| IBIS file stm32u535_545_wlcsp72.ibs
[IBIS ver] 4.2
[File name] stm32u535_545_wlcsp72.ibs
[File Rev] rev1.0
[Date]  11-09-2023
[Source] Data Created at STMicroelectronics
[Notes]  File originated from ELDO simulations.
[Disclaimer]  This information is for modeling purpose only and is
   not guaranteed. The information is subject to change without
   notice.
[Copyright] Copyright 2023 STMicroelectronics Inc.
|   Component stm32u535_545_wlcsp72
[Component] stm32u535_545_wlcsp72
[Manufacturer] STMicroelectronics
[Package]
| variable   typ   min   max
R_pkg  0  NA  NA
L_pkg  0  NA  NA
C_pkg  0  NA  NA
[Pin]   signal_name   model_name
A2  VDD  power
A4  PG10  io8_100m_hslv_ft
A6  PG14  io8_100m_hslv_i2c_ft
A8  VDDIO2  power
A10  PB4  io8_100m_i2c_ft
A12  PH3-BOOT0  io8_100m_ft
A14  VDD11  nc
A16  VDD  power
B1  VDDUSB  power
B3  VSS  gnd
B5  PG9  io8_100m_hslv_ft
B7  VSS  gnd
B9  PG15  io8_100m_hslv_ft
B11  PB6  io8_100m_i2c_ft
B13  VSS  gnd
B15  VBAT  power
C2  PA11  io8_usb_ft
C4  PA12  io8_usb_ft
C6  PG11  io8_100m_hslv_ft
C8  PG13  io8_100m_hslv_i2c_ft
C10  PB3  io8_100m_i2c_ft
C12  PB8  io8_100m_hslv_i2c_ft
C14  PC13  io8_100m_ft_v33
C16  PC14-OSC32_IN   io8_100m_tamp_ft
D1  VDDIO2  power
D3  VSS  gnd
D5  PA13  io8_100m_ft
D7  PA15  io8_100m_ft
D9  PG12  io8_100m_hslv_ft
D11  PB5  io8_166m_hslv_ft
D13  PB7  io8_166m_hslv_i2c_ft
D15  PC15-OSC32_OUT  io8_100m_tamp_ft
E2  PG8  io8_100m_i2c_ft
E4  PA8  io8_166m_hslv_ft
E6  PA10  io8_100m_ft
E8  PA14  io8_100m_ft
E10  PA5  io8_100m_ft
E12  PA1  io8_100m_hslv_tamp_ft
E14  NRST  nc
E16  PH0-OSC_IN  io8_100m_ft
F1  PG4  io8_100m_hslv_ft
F3  PG5  io8_100m_hslv_ft
F5  PG6  io8_100m_hslv_ft
F7  PG7  io8_100m_hslv_i2c_ft
F9  PA9  io8_100m_ft
F11  PA2  io8_100m_hslv_ft
F13  PC1  io8_166m_hslv_i2c_ft
F15  PH1-OSC_OUT  io8_100m_ft
G2  PB14  io8_100m_i2c_ft
G4  PB13  io8_100m_i2c_ft
G6  PG2  io8_100m_hslv_ft
G8  PB1  io8_100m_hslv_ft
G10  PB0  io8_100m_hslv_ft
G12  PA3  io8_166m_hslv_ft
G14  VDDA  power
G16  VSSA  nc
H1  PB15  io8_100m_ft
H3  VSS  gnd
H5  VSSSMPS  nc
H7  PG3  io8_100m_hslv_ft
H9  PB10  io8_166m_hslv_i2c_ft
H11  PA6  io8_100m_hslv_ft
H13  PA4  io8_100m_hslv_ft
H15  PA0  io8_100m_hslv_tamp_ft
J2  VDD  power
J4  VDD11  nc
J6  VDDSMPS  nc
J8  VLXSMPS  nc
J10  PB2  io8_100m_hslv_tamp_ft
J12  PA7  io8_100m_hslv_i2c_ft
J14  VDD  power
J16  VSS  gnd
[Package Model]   455-wlcsp-72-100mhz-230421
[Pin Mapping]   pulldown_ref   pullup_ref   | Comment
A2  nc  vddiom
A4  gndio  vddiom
A6  gndio  vddiom  | Depending on IO usage
| A6  gndio  vddios  | Depending on IO usage
A8  nc  vddios
A10  gndio  vddiom
A12  gndio  vddiom
A14  nc  nc
A16  nc  vddiom
B1  nc  vddusb
B3  gndio  nc
B5  gndio  vddiom  | Depending on IO usage
| B5  gndio  vddios  | Depending on IO usage
B7  gndio  nc
B9  gndio  vddiom  | Depending on IO usage
| B9  gndio  vddios  | Depending on IO usage
B11  gndio  vddiom
B13  gndio  nc
B15  nc  vsw
C2  gndio  vddiom  | Depending on IO usage
| C2  gndio  vddusb  | Depending on IO usage
C4  gndio  vddiom  | Depending on IO usage
| C4  gndio  vddusb  | Depending on IO usage
C6  gndio  vddiom  | Depending on IO usage
| C6  gndio  vddios  | Depending on IO usage
C8  gndio  vddiom  | Depending on IO usage
| C8  gndio  vddios  | Depending on IO usage
C10  gndio  vddiom
C12  gndio  vddiom
C14  gndio  vddiom  | Depending on IO usage
| C14  gndio  vsw  | Depending on IO usage
C16  gndio  vddiom  | Depending on IO usage
| C16  gndio  vsw  | Depending on IO usage
D1  nc  vddios
D3  gndio  nc
D5  gndio  vddiom  | Depending on IO usage
| D5  gndio  vddusb  | Depending on IO usage
D7  gndio  vddiom
D9  gndio  vddiom  | Depending on IO usage
| D9  gndio  vddios  | Depending on IO usage
D11  gndio  vddiom
D13  gndio  vddiom
D15  gndio  vddiom  | Depending on IO usage
| D15  gndio  vsw  | Depending on IO usage
E2  gndio  vddiom  | Depending on IO usage
| E2  gndio  vddios  | Depending on IO usage
E4  gndio  vddiom
E6  gndio  vddiom  | Depending on IO usage
| E6  gndio  vddusb  | Depending on IO usage
E8  gndio  vddiom
E10  gndio  vddiom
E12  gndio  vddiom
E14  nc   nc
E16  gndio  vddiom
F1  gndio  vddiom  | Depending on IO usage
| F1  gndio  vddios  | Depending on IO usage
F3  gndio  vddiom  | Depending on IO usage
| F3  gndio  vddios  | Depending on IO usage
F5  gndio  vddiom  | Depending on IO usage
| F5  gndio  vddios  | Depending on IO usage
F7  gndio  vddiom  | Depending on IO usage
| F7  gndio  vddios  | Depending on IO usage
F9  gndio  vddiom  | Depending on IO usage
| F9  gndio  vddusb  | Depending on IO usage
F11  gndio  vddiom
F13  gndio  vddiom
F15  gndio  vddiom
G2  gndio  vddiom
G4  gndio  vddiom
G6  gndio  vddiom  | Depending on IO usage
| G6  gndio  vddios  | Depending on IO usage
G8  gndio  vddiom
G10  gndio  vddiom
G12  gndio  vddiom
G14  nc  vddiom
G16  nc  nc
H1  gndio  vddiom
H3  gndio  nc
H5  nc  nc
H7  gndio  vddiom  | Depending on IO usage
| H7  gndio  vddios  | Depending on IO usage
H9  gndio  vddiom
H11  gndio  vddiom
H13  gndio  vddiom
H15  gndio  vddiom
J2  nc  vddiom
J4  nc  nc
J6  nc  nc
J8  nc  nc
J10  gndio  vddiom
J12  gndio  vddiom
J14  nc  vddiom
J16  gndio  nc
[Model Selector] io8_100m_ft
io8_100m_ft_hs_1v2  "IO8_FT 100MHz high speed @ 1.2V"
io8_100m_ft_fs_1v2  "IO8_FT 100MHz fast speed @ 1.2V"
io8_100m_ft_fs_pd_1v2  "IO8_FT 100MHz fast speed @ 1.2V pulldown"
io8_100m_ft_ms_1v2  "IO8_FT 100MHz med speed @ 1.2V"
io8_100m_ft_ms_pd_1v2  "IO8_FT 100MHz med speed @ 1.2V pulldown"
io8_100m_ft_ls_1v2  "IO8_FT 100MHz low speed @ 1.2V"
io8_100m_ft_ls_pd_1v2  "IO8_FT 100MHz low speed @ 1.2V pulldown"
io8_100m_ft_hs_1v8  "IO8_FT 100MHz high speed @ 1.8V"
io8_100m_ft_hs_pd_1v8  "IO8_FT 100MHz high speed @ 1.8V pulldown"
io8_100m_ft_fs_1v8  "IO8_FT 100MHz fast speed @ 1.8V"
io8_100m_ft_fs_pd_1v8  "IO8_FT 100MHz fast speed @ 1.8V pulldown"
io8_100m_ft_ms_1v8  "IO8_FT 100MHz med speed @ 1.8V"
io8_100m_ft_ms_pd_1v8  "IO8_FT 100MHz med speed @ 1.8V pulldown"
io8_100m_ft_ls_1v8  "IO8_FT 100MHz low speed @ 1.8V"
io8_100m_ft_ls_pd_1v8  "IO8_FT 100MHz low speed @ 1.8V pulldown"
io8_100m_ft_hs_3v3  "IO8_FT 100MHz high speed @ 3.3V"
io8_100m_ft_hs_pd_3v3  "IO8_FT 100MHz high speed @ 3.3V pulldown"
io8_100m_ft_fs_3v3  "IO8_FT 100MHz fast speed @ 3.3V"
io8_100m_ft_fs_pd_3v3  "IO8_FT 100MHz fast speed @ 3.3V pulldown"
io8_100m_ft_ms_3v3  "IO8_FT 100MHz med speed @ 3.3V"
io8_100m_ft_ms_pd_3v3  "IO8_FT 100MHz med speed @ 3.3V pulldown"
io8_100m_ft_ls_3v3  "IO8_FT 100MHz low speed @ 3.3V"
io8_100m_ft_ls_pd_3v3  "IO8_FT 100MHz low speed @ 3.3V pulldown"
[Model Selector] io8_100m_hslv_ft
io8_100m_ft_hs_1v2  "IO8_FT 100MHz high speed @ 1.2V"
io8_100m_ft_hs_pu_1v2  "IO8_FT 100MHz high speed @ 1.2V pullup"
io8_100m_ft_hs_pd_1v2  "IO8_FT 100MHz high speed @ 1.2V pulldown"
io8_100m_ft_fs_1v2  "IO8_FT 100MHz fast speed @ 1.2V"
io8_100m_ft_fs_pu_1v2  "IO8_FT 100MHz fast speed @ 1.2V pullup"
io8_100m_ft_fs_pd_1v2  "IO8_FT 100MHz fast speed @ 1.2V pulldown"
io8_100m_ft_ms_1v2  "IO8_FT 100MHz med speed @ 1.2V"
io8_100m_ft_ms_pu_1v2  "IO8_FT 100MHz med speed @ 1.2V pullup"
io8_100m_ft_ms_pd_1v2  "IO8_FT 100MHz med speed @ 1.2V pulldown"
io8_100m_ft_ls_1v2  "IO8_FT 100MHz low speed @ 1.2V"
io8_100m_ft_ls_pu_1v2  "IO8_FT 100MHz low speed @ 1.2V pullup"
io8_100m_ft_ls_pd_1v2  "IO8_FT 100MHz low speed @ 1.2V pulldown"
io8_100m_ft_hs_1v8  "IO8_FT 100MHz high speed @ 1.8V"
io8_100m_ft_hs_pu_1v8  "IO8_FT 100MHz high speed @ 1.8V pullup"
io8_100m_ft_hs_pd_1v8  "IO8_FT 100MHz high speed @ 1.8V pulldown"
io8_100m_ft_fs_1v8  "IO8_FT 100MHz fast speed @ 1.8V"
io8_100m_ft_fs_pu_1v8  "IO8_FT 100MHz fast speed @ 1.8V pullup"
io8_100m_ft_fs_pd_1v8  "IO8_FT 100MHz fast speed @ 1.8V pulldown"
io8_100m_ft_ms_1v8  "IO8_FT 100MHz med speed @ 1.8V"
io8_100m_ft_ms_pu_1v8  "IO8_FT 100MHz med speed @ 1.8V pullup"
io8_100m_ft_ms_pd_1v8  "IO8_FT 100MHz med speed @ 1.8V pulldown"
io8_100m_ft_ls_1v8  "IO8_FT 100MHz low speed @ 1.8V"
io8_100m_ft_ls_pu_1v8  "IO8_FT 100MHz low speed @ 1.8V pullup"
io8_100m_ft_ls_pd_1v8  "IO8_FT 100MHz low speed @ 1.8V pulldown"
io8_100m_ft_hs_3v3  "IO8_FT 100MHz high speed @ 3.3V"
io8_100m_ft_hs_pu_3v3  "IO8_FT 100MHz high speed @ 3.3V pullup"
io8_100m_ft_hs_pd_3v3  "IO8_FT 100MHz high speed @ 3.3V pulldown"
io8_100m_ft_fs_3v3  "IO8_FT 100MHz fast speed @ 3.3V"
io8_100m_ft_fs_pu_3v3  "IO8_FT 100MHz fast speed @ 3.3V pullup"
io8_100m_ft_fs_pd_3v3  "IO8_FT 100MHz fast speed @ 3.3V pulldown"
io8_100m_ft_ms_3v3  "IO8_FT 100MHz med speed @ 3.3V"
io8_100m_ft_ms_pu_3v3  "IO8_FT 100MHz med speed @ 3.3V pullup"
io8_100m_ft_ms_pd_3v3  "IO8_FT 100MHz med speed @ 3.3V pulldown"
io8_100m_ft_ls_3v3  "IO8_FT 100MHz low speed @ 3.3V"
io8_100m_ft_ls_pu_3v3  "IO8_FT 100MHz low speed @ 3.3V pullup"
io8_100m_ft_ls_pd_3v3  "IO8_FT 100MHz low speed @ 3.3V pulldown"
io8_100m_hslv_ft_hs_1v2  "IO8_FT 100MHz HSLV high speed @ 1.2V"
io8_100m_hslv_ft_hs_pu_1v2  "IO8_FT 100MHz HSLV high speed @ 1.2V pullup"
io8_100m_hslv_ft_hs_pd_1v2  "IO8_FT 100MHz HSLV high speed @ 1.2V pulldown"
io8_100m_hslv_ft_fs_1v2  "IO8_FT 100MHz HSLV fast speed @ 1.2V"
io8_100m_hslv_ft_fs_pu_1v2  "IO8_FT 100MHz HSLV fast speed @ 1.2V pullup"
io8_100m_hslv_ft_fs_pd_1v2  "IO8_FT 100MHz HSLV fast speed @ 1.2V pulldown"
io8_100m_hslv_ft_ms_1v2  "IO8_FT 100MHz HSLV med speed @ 1.2V"
io8_100m_hslv_ft_ms_pu_1v2  "IO8_FT 100MHz HSLV med speed @ 1.2V pullup"
io8_100m_hslv_ft_ms_pd_1v2  "IO8_FT 100MHz HSLV med speed @ 1.2V pulldown"
io8_100m_hslv_ft_ls_1v2  "IO8_FT 100MHz HSLV low speed @ 1.2V"
io8_100m_hslv_ft_ls_pu_1v2  "IO8_FT 100MHz HSLV low speed @ 1.2V pullup"
io8_100m_hslv_ft_ls_pd_1v2  "IO8_FT 100MHz HSLV low speed @ 1.2V pulldown"
io8_100m_hslv_ft_hs_1v8  "IO8_FT 100MHz HSLV high speed @ 1.8V"
io8_100m_hslv_ft_hs_pu_1v8  "IO8_FT 100MHz HSLV high speed @ 1.8V pullup"
io8_100m_hslv_ft_hs_pd_1v8  "IO8_FT 100MHz HSLV high speed @ 1.8V pulldown"
io8_100m_hslv_ft_fs_1v8  "IO8_FT 100MHz HSLV fast speed @ 1.8V"
io8_100m_hslv_ft_fs_pu_1v8  "IO8_FT 100MHz HSLV fast speed @ 1.8V pullup"
io8_100m_hslv_ft_fs_pd_1v8  "IO8_FT 100MHz HSLV fast speed @ 1.8V pulldown"
io8_100m_hslv_ft_ms_1v8  "IO8_FT 100MHz HSLV med speed @ 1.8V"
io8_100m_hslv_ft_ms_pu_1v8  "IO8_FT 100MHz HSLV med speed @ 1.8V pullup"
io8_100m_hslv_ft_ms_pd_1v8  "IO8_FT 100MHz HSLV med speed @ 1.8V pulldown"
io8_100m_hslv_ft_ls_1v8  "IO8_FT 100MHz HSLV low speed @ 1.8V"
io8_100m_hslv_ft_ls_pu_1v8  "IO8_FT 100MHz HSLV low speed @ 1.8V pullup"
io8_100m_hslv_ft_ls_pd_1v8  "IO8_FT 100MHz HSLV low speed @ 1.8V pulldown"
io8_100m_hslv_ft_hs_2v5  "IO8_FT 100MHz HSLV high speed @ 2.5V"
io8_100m_hslv_ft_hs_pu_2v5  "IO8_FT 100MHz HSLV high speed @ 2.5V pullup"
io8_100m_hslv_ft_hs_pd_2v5  "IO8_FT 100MHz HSLV high speed @ 2.5V pulldown"
io8_100m_hslv_ft_fs_2v5  "IO8_FT 100MHz HSLV fast speed @ 2.5V"
io8_100m_hslv_ft_fs_pu_2v5  "IO8_FT 100MHz HSLV fast speed @ 2.5V pullup"
io8_100m_hslv_ft_fs_pd_2v5  "IO8_FT 100MHz HSLV fast speed @ 2.5V pulldown"
io8_100m_hslv_ft_ms_2v5  "IO8_FT 100MHz HSLV med speed @ 2.5V"
io8_100m_hslv_ft_ms_pu_2v5  "IO8_FT 100MHz HSLV med speed @ 2.5V pullup"
io8_100m_hslv_ft_ms_pd_2v5  "IO8_FT 100MHz HSLV med speed @ 2.5V pulldown"
io8_100m_hslv_ft_ls_2v5  "IO8_FT 100MHz HSLV low speed @ 2.5V"
io8_100m_hslv_ft_ls_pu_2v5  "IO8_FT 100MHz HSLV low speed @ 2.5V pullup"
io8_100m_hslv_ft_ls_pd_2v5  "IO8_FT 100MHz HSLV low speed @ 2.5V pulldown"
[Model Selector] io8_100m_hslv_i2c_ft
io8_100m_ft_hs_1v2  "IO8_FT 100MHz high speed @ 1.2V"
io8_100m_ft_hs_pu_1v2  "IO8_FT 100MHz high speed @ 1.2V pullup"
io8_100m_ft_hs_pd_1v2  "IO8_FT 100MHz high speed @ 1.2V pulldown"
io8_100m_ft_fs_1v2  "IO8_FT 100MHz fast speed @ 1.2V"
io8_100m_ft_fs_pu_1v2  "IO8_FT 100MHz fast speed @ 1.2V pullup"
io8_100m_ft_fs_pd_1v2  "IO8_FT 100MHz fast speed @ 1.2V pulldown"
io8_100m_ft_ms_1v2  "IO8_FT 100MHz med speed @ 1.2V"
io8_100m_ft_ms_pu_1v2  "IO8_FT 100MHz med speed @ 1.2V pullup"
io8_100m_ft_ms_pd_1v2  "IO8_FT 100MHz med speed @ 1.2V pulldown"
io8_100m_ft_ls_1v2  "IO8_FT 100MHz low speed @ 1.2V"
io8_100m_ft_ls_pu_1v2  "IO8_FT 100MHz low speed @ 1.2V pullup"
io8_100m_ft_ls_pd_1v2  "IO8_FT 100MHz low speed @ 1.2V pulldown"
io8_100m_ft_hs_1v8  "IO8_FT 100MHz high speed @ 1.8V"
io8_100m_ft_hs_pu_1v8  "IO8_FT 100MHz high speed @ 1.8V pullup"
io8_100m_ft_hs_pd_1v8  "IO8_FT 100MHz high speed @ 1.8V pulldown"
io8_100m_ft_fs_1v8  "IO8_FT 100MHz fast speed @ 1.8V"
io8_100m_ft_fs_pu_1v8  "IO8_FT 100MHz fast speed @ 1.8V pullup"
io8_100m_ft_fs_pd_1v8  "IO8_FT 100MHz fast speed @ 1.8V pulldown"
io8_100m_ft_ms_1v8  "IO8_FT 100MHz med speed @ 1.8V"
io8_100m_ft_ms_pu_1v8  "IO8_FT 100MHz med speed @ 1.8V pullup"
io8_100m_ft_ms_pd_1v8  "IO8_FT 100MHz med speed @ 1.8V pulldown"
io8_100m_ft_ls_1v8  "IO8_FT 100MHz low speed @ 1.8V"
io8_100m_ft_ls_pu_1v8  "IO8_FT 100MHz low speed @ 1.8V pullup"
io8_100m_ft_ls_pd_1v8  "IO8_FT 100MHz low speed @ 1.8V pulldown"
io8_100m_ft_hs_3v3  "IO8_FT 100MHz high speed @ 3.3V"
io8_100m_ft_hs_pu_3v3  "IO8_FT 100MHz high speed @ 3.3V pullup"
io8_100m_ft_hs_pd_3v3  "IO8_FT 100MHz high speed @ 3.3V pulldown"
io8_100m_ft_fs_3v3  "IO8_FT 100MHz fast speed @ 3.3V"
io8_100m_ft_fs_pu_3v3  "IO8_FT 100MHz fast speed @ 3.3V pullup"
io8_100m_ft_fs_pd_3v3  "IO8_FT 100MHz fast speed @ 3.3V pulldown"
io8_100m_ft_ms_3v3  "IO8_FT 100MHz med speed @ 3.3V"
io8_100m_ft_ms_pu_3v3  "IO8_FT 100MHz med speed @ 3.3V pullup"
io8_100m_ft_ms_pd_3v3  "IO8_FT 100MHz med speed @ 3.3V pulldown"
io8_100m_ft_ls_3v3  "IO8_FT 100MHz low speed @ 3.3V"
io8_100m_ft_ls_pu_3v3  "IO8_FT 100MHz low speed @ 3.3V pullup"
io8_100m_ft_ls_pd_3v3  "IO8_FT 100MHz low speed @ 3.3V pulldown"
io8_100m_hslv_ft_hs_1v2  "IO8_FT 100MHz HSLV high speed @ 1.2V"
io8_100m_hslv_ft_hs_pu_1v2  "IO8_FT 100MHz HSLV high speed @ 1.2V pullup"
io8_100m_hslv_ft_hs_pd_1v2  "IO8_FT 100MHz HSLV high speed @ 1.2V pulldown"
io8_100m_hslv_ft_fs_1v2  "IO8_FT 100MHz HSLV fast speed @ 1.2V"
io8_100m_hslv_ft_fs_pu_1v2  "IO8_FT 100MHz HSLV fast speed @ 1.2V pullup"
io8_100m_hslv_ft_fs_pd_1v2  "IO8_FT 100MHz HSLV fast speed @ 1.2V pulldown"
io8_100m_hslv_ft_ms_1v2  "IO8_FT 100MHz HSLV med speed @ 1.2V"
io8_100m_hslv_ft_ms_pu_1v2  "IO8_FT 100MHz HSLV med speed @ 1.2V pullup"
io8_100m_hslv_ft_ms_pd_1v2  "IO8_FT 100MHz HSLV med speed @ 1.2V pulldown"
io8_100m_hslv_ft_ls_1v2  "IO8_FT 100MHz HSLV low speed @ 1.2V"
io8_100m_hslv_ft_ls_pu_1v2  "IO8_FT 100MHz HSLV low speed @ 1.2V pullup"
io8_100m_hslv_ft_ls_pd_1v2  "IO8_FT 100MHz HSLV low speed @ 1.2V pulldown"
io8_100m_hslv_ft_hs_1v8  "IO8_FT 100MHz HSLV high speed @ 1.8V"
io8_100m_hslv_ft_hs_pu_1v8  "IO8_FT 100MHz HSLV high speed @ 1.8V pullup"
io8_100m_hslv_ft_hs_pd_1v8  "IO8_FT 100MHz HSLV high speed @ 1.8V pulldown"
io8_100m_hslv_ft_fs_1v8  "IO8_FT 100MHz HSLV fast speed @ 1.8V"
io8_100m_hslv_ft_fs_pu_1v8  "IO8_FT 100MHz HSLV fast speed @ 1.8V pullup"
io8_100m_hslv_ft_fs_pd_1v8  "IO8_FT 100MHz HSLV fast speed @ 1.8V pulldown"
io8_100m_hslv_ft_ms_1v8  "IO8_FT 100MHz HSLV med speed @ 1.8V"
io8_100m_hslv_ft_ms_pu_1v8  "IO8_FT 100MHz HSLV med speed @ 1.8V pullup"
io8_100m_hslv_ft_ms_pd_1v8  "IO8_FT 100MHz HSLV med speed @ 1.8V pulldown"
io8_100m_hslv_ft_ls_1v8  "IO8_FT 100MHz HSLV low speed @ 1.8V"
io8_100m_hslv_ft_ls_pu_1v8  "IO8_FT 100MHz HSLV low speed @ 1.8V pullup"
io8_100m_hslv_ft_ls_pd_1v8  "IO8_FT 100MHz HSLV low speed @ 1.8V pulldown"
io8_100m_hslv_ft_hs_2v5  "IO8_FT 100MHz HSLV high speed @ 2.5V"
io8_100m_hslv_ft_hs_pu_2v5  "IO8_FT 100MHz HSLV high speed @ 2.5V pullup"
io8_100m_hslv_ft_hs_pd_2v5  "IO8_FT 100MHz HSLV high speed @ 2.5V pulldown"
io8_100m_hslv_ft_fs_2v5  "IO8_FT 100MHz HSLV fast speed @ 2.5V"
io8_100m_hslv_ft_fs_pu_2v5  "IO8_FT 100MHz HSLV fast speed @ 2.5V pullup"
io8_100m_hslv_ft_fs_pd_2v5  "IO8_FT 100MHz HSLV fast speed @ 2.5V pulldown"
io8_100m_hslv_ft_ms_2v5  "IO8_FT 100MHz HSLV med speed @ 2.5V"
io8_100m_hslv_ft_ms_pu_2v5  "IO8_FT 100MHz HSLV med speed @ 2.5V pullup"
io8_100m_hslv_ft_ms_pd_2v5  "IO8_FT 100MHz HSLV med speed @ 2.5V pulldown"
io8_100m_hslv_ft_ls_2v5  "IO8_FT 100MHz HSLV low speed @ 2.5V"
io8_100m_hslv_ft_ls_pu_2v5  "IO8_FT 100MHz HSLV low speed @ 2.5V pullup"
io8_100m_hslv_ft_ls_pd_2v5  "IO8_FT 100MHz HSLV low speed @ 2.5V pulldown"
[Model Selector] io8_100m_hslv_tamp_ft
io8_100m_ft_hs_1v2  "IO8_FT 100MHz high speed @ 1.2V"
io8_100m_ft_hs_pu_1v2  "IO8_FT 100MHz high speed @ 1.2V pullup"
io8_100m_ft_hs_pd_1v2  "IO8_FT 100MHz high speed @ 1.2V pulldown"
io8_100m_ft_fs_1v2  "IO8_FT 100MHz fast speed @ 1.2V"
io8_100m_ft_fs_pu_1v2  "IO8_FT 100MHz fast speed @ 1.2V pullup"
io8_100m_ft_fs_pd_1v2  "IO8_FT 100MHz fast speed @ 1.2V pulldown"
io8_100m_ft_ms_1v2  "IO8_FT 100MHz med speed @ 1.2V"
io8_100m_ft_ms_pu_1v2  "IO8_FT 100MHz med speed @ 1.2V pullup"
io8_100m_ft_ms_pd_1v2  "IO8_FT 100MHz med speed @ 1.2V pulldown"
io8_100m_ft_ls_1v2  "IO8_FT 100MHz low speed @ 1.2V"
io8_100m_ft_ls_pu_1v2  "IO8_FT 100MHz low speed @ 1.2V pullup"
io8_100m_ft_ls_pd_1v2  "IO8_FT 100MHz low speed @ 1.2V pulldown"
io8_100m_ft_hs_1v8  "IO8_FT 100MHz high speed @ 1.8V"
io8_100m_ft_hs_pu_1v8  "IO8_FT 100MHz high speed @ 1.8V pullup"
io8_100m_ft_hs_pd_1v8  "IO8_FT 100MHz high speed @ 1.8V pulldown"
io8_100m_ft_fs_1v8  "IO8_FT 100MHz fast speed @ 1.8V"
io8_100m_ft_fs_pu_1v8  "IO8_FT 100MHz fast speed @ 1.8V pullup"
io8_100m_ft_fs_pd_1v8  "IO8_FT 100MHz fast speed @ 1.8V pulldown"
io8_100m_ft_ms_1v8  "IO8_FT 100MHz med speed @ 1.8V"
io8_100m_ft_ms_pu_1v8  "IO8_FT 100MHz med speed @ 1.8V pullup"
io8_100m_ft_ms_pd_1v8  "IO8_FT 100MHz med speed @ 1.8V pulldown"
io8_100m_ft_ls_1v8  "IO8_FT 100MHz low speed @ 1.8V"
io8_100m_ft_ls_pu_1v8  "IO8_FT 100MHz low speed @ 1.8V pullup"
io8_100m_ft_ls_pd_1v8  "IO8_FT 100MHz low speed @ 1.8V pulldown"
io8_100m_ft_hs_3v3  "IO8_FT 100MHz high speed @ 3.3V"
io8_100m_ft_hs_pu_3v3  "IO8_FT 100MHz high speed @ 3.3V pullup"
io8_100m_ft_hs_pd_3v3  "IO8_FT 100MHz high speed @ 3.3V pulldown"
io8_100m_ft_fs_3v3  "IO8_FT 100MHz fast speed @ 3.3V"
io8_100m_ft_fs_pu_3v3  "IO8_FT 100MHz fast speed @ 3.3V pullup"
io8_100m_ft_fs_pd_3v3  "IO8_FT 100MHz fast speed @ 3.3V pulldown"
io8_100m_ft_ms_3v3  "IO8_FT 100MHz med speed @ 3.3V"
io8_100m_ft_ms_pu_3v3  "IO8_FT 100MHz med speed @ 3.3V pullup"
io8_100m_ft_ms_pd_3v3  "IO8_FT 100MHz med speed @ 3.3V pulldown"
io8_100m_ft_ls_3v3  "IO8_FT 100MHz low speed @ 3.3V"
io8_100m_ft_ls_pu_3v3  "IO8_FT 100MHz low speed @ 3.3V pullup"
io8_100m_ft_ls_pd_3v3  "IO8_FT 100MHz low speed @ 3.3V pulldown"
io8_100m_hslv_ft_hs_1v2  "IO8_FT 100MHz HSLV high speed @ 1.2V"
io8_100m_hslv_ft_hs_pu_1v2  "IO8_FT 100MHz HSLV high speed @ 1.2V pullup"
io8_100m_hslv_ft_hs_pd_1v2  "IO8_FT 100MHz HSLV high speed @ 1.2V pulldown"
io8_100m_hslv_ft_fs_1v2  "IO8_FT 100MHz HSLV fast speed @ 1.2V"
io8_100m_hslv_ft_fs_pu_1v2  "IO8_FT 100MHz HSLV fast speed @ 1.2V pullup"
io8_100m_hslv_ft_fs_pd_1v2  "IO8_FT 100MHz HSLV fast speed @ 1.2V pulldown"
io8_100m_hslv_ft_ms_1v2  "IO8_FT 100MHz HSLV med speed @ 1.2V"
io8_100m_hslv_ft_ms_pu_1v2  "IO8_FT 100MHz HSLV med speed @ 1.2V pullup"
io8_100m_hslv_ft_ms_pd_1v2  "IO8_FT 100MHz HSLV med speed @ 1.2V pulldown"
io8_100m_hslv_ft_ls_1v2  "IO8_FT 100MHz HSLV low speed @ 1.2V"
io8_100m_hslv_ft_ls_pu_1v2  "IO8_FT 100MHz HSLV low speed @ 1.2V pullup"
io8_100m_hslv_ft_ls_pd_1v2  "IO8_FT 100MHz HSLV low speed @ 1.2V pulldown"
io8_100m_hslv_ft_hs_1v8  "IO8_FT 100MHz HSLV high speed @ 1.8V"
io8_100m_hslv_ft_hs_pu_1v8  "IO8_FT 100MHz HSLV high speed @ 1.8V pullup"
io8_100m_hslv_ft_hs_pd_1v8  "IO8_FT 100MHz HSLV high speed @ 1.8V pulldown"
io8_100m_hslv_ft_fs_1v8  "IO8_FT 100MHz HSLV fast speed @ 1.8V"
io8_100m_hslv_ft_fs_pu_1v8  "IO8_FT 100MHz HSLV fast speed @ 1.8V pullup"
io8_100m_hslv_ft_fs_pd_1v8  "IO8_FT 100MHz HSLV fast speed @ 1.8V pulldown"
io8_100m_hslv_ft_ms_1v8  "IO8_FT 100MHz HSLV med speed @ 1.8V"
io8_100m_hslv_ft_ms_pu_1v8  "IO8_FT 100MHz HSLV med speed @ 1.8V pullup"
io8_100m_hslv_ft_ms_pd_1v8  "IO8_FT 100MHz HSLV med speed @ 1.8V pulldown"
io8_100m_hslv_ft_ls_1v8  "IO8_FT 100MHz HSLV low speed @ 1.8V"
io8_100m_hslv_ft_ls_pu_1v8  "IO8_FT 100MHz HSLV low speed @ 1.8V pullup"
io8_100m_hslv_ft_ls_pd_1v8  "IO8_FT 100MHz HSLV low speed @ 1.8V pulldown"
io8_100m_hslv_ft_hs_2v5  "IO8_FT 100MHz HSLV high speed @ 2.5V"
io8_100m_hslv_ft_hs_pu_2v5  "IO8_FT 100MHz HSLV high speed @ 2.5V pullup"
io8_100m_hslv_ft_hs_pd_2v5  "IO8_FT 100MHz HSLV high speed @ 2.5V pulldown"
io8_100m_hslv_ft_fs_2v5  "IO8_FT 100MHz HSLV fast speed @ 2.5V"
io8_100m_hslv_ft_fs_pu_2v5  "IO8_FT 100MHz HSLV fast speed @ 2.5V pullup"
io8_100m_hslv_ft_fs_pd_2v5  "IO8_FT 100MHz HSLV fast speed @ 2.5V pulldown"
io8_100m_hslv_ft_ms_2v5  "IO8_FT 100MHz HSLV med speed @ 2.5V"
io8_100m_hslv_ft_ms_pu_2v5  "IO8_FT 100MHz HSLV med speed @ 2.5V pullup"
io8_100m_hslv_ft_ms_pd_2v5  "IO8_FT 100MHz HSLV med speed @ 2.5V pulldown"
io8_100m_hslv_ft_ls_2v5  "IO8_FT 100MHz HSLV low speed @ 2.5V"
io8_100m_hslv_ft_ls_pu_2v5  "IO8_FT 100MHz HSLV low speed @ 2.5V pullup"
io8_100m_hslv_ft_ls_pd_2v5  "IO8_FT 100MHz HSLV low speed @ 2.5V pulldown"
io8_ft_v33_hs_1v2  "IO8_FT_V33 high speed @ 1.2V"
io8_ft_v33_hs_pu_1v2  "IO8_FT_V33 high speed @ 1.2V pullup"
io8_ft_v33_hs_pd_1v2  "IO8_FT_V33 high speed @ 1.2V pulldown"
io8_ft_v33_fs_1v2  "IO8_FT_V33 fast speed @ 1.2V"
io8_ft_v33_fs_pu_1v2  "IO8_FT_V33 fast speed @ 1.2V pullup"
io8_ft_v33_fs_pd_1v2  "IO8_FT_V33 fast speed @ 1.2V pulldown"
io8_ft_v33_ms_1v2  "IO8_FT_V33 med speed @ 1.2V"
io8_ft_v33_ms_pu_1v2  "IO8_FT_V33 med speed @ 1.2V pullup"
io8_ft_v33_ms_pd_1v2  "IO8_FT_V33 med speed @ 1.2V pulldown"
io8_ft_v33_ls_1v2  "IO8_FT_V33 low speed @ 1.2V"
io8_ft_v33_ls_pu_1v2  "IO8_FT_V33 low speed @ 1.2V pullup"
io8_ft_v33_ls_pd_1v2  "IO8_FT_V33 low speed @ 1.2V pulldown"
io8_ft_v33_hs_1v8  "IO8_FT_V33 high speed @ 1.8V"
io8_ft_v33_hs_pu_1v8  "IO8_FT_V33 high speed @ 1.8V pullup"
io8_ft_v33_hs_pd_1v8  "IO8_FT_V33 high speed @ 1.8V pulldown"
io8_ft_v33_fs_1v8  "IO8_FT_V33 fast speed @ 1.8V"
io8_ft_v33_fs_pu_1v8  "IO8_FT_V33 fast speed @ 1.8V pullup"
io8_ft_v33_fs_pd_1v8  "IO8_FT_V33 fast speed @ 1.8V pulldown"
io8_ft_v33_ms_1v8  "IO8_FT_V33 med speed @ 1.8V"
io8_ft_v33_ms_pu_1v8  "IO8_FT_V33 med speed @ 1.8V pullup"
io8_ft_v33_ms_pd_1v8  "IO8_FT_V33 med speed @ 1.8V pulldown"
io8_ft_v33_ls_1v8  "IO8_FT_V33 low speed @ 1.8V"
io8_ft_v33_ls_pu_1v8  "IO8_FT_V33 low speed @ 1.8V pullup"
io8_ft_v33_ls_pd_1v8  "IO8_FT_V33 low speed @ 1.8V pulldown"
io8_ft_v33_hs_3v3  "IO8_FT_V33 high speed @ 3.3V"
io8_ft_v33_hs_pu_3v3  "IO8_FT_V33 high speed @ 3.3V pullup"
io8_ft_v33_hs_pd_3v3  "IO8_FT_V33 high speed @ 3.3V pulldown"
io8_ft_v33_fs_3v3  "IO8_FT_V33 fast speed @ 3.3V"
io8_ft_v33_fs_pu_3v3  "IO8_FT_V33 fast speed @ 3.3V pullup"
io8_ft_v33_fs_pd_3v3  "IO8_FT_V33 fast speed @ 3.3V pulldown"
io8_ft_v33_ms_3v3  "IO8_FT_V33 med speed @ 3.3V"
io8_ft_v33_ms_pu_3v3  "IO8_FT_V33 med speed @ 3.3V pullup"
io8_ft_v33_ms_pd_3v3  "IO8_FT_V33 med speed @ 3.3V pulldown"
io8_ft_v33_ls_3v3  "IO8_FT_V33 low speed @ 3.3V"
io8_ft_v33_ls_pu_3v3  "IO8_FT_V33 low speed @ 3.3V pullup"
io8_ft_v33_ls_pd_3v3  "IO8_FT_V33 low speed @ 3.3V pulldown"
[Model Selector] io8_100m_i2c_ft
io8_100m_ft_hs_1v2  "IO8_FT 100MHz high speed @ 1.2V"
io8_100m_ft_hs_pu_1v2  "IO8_FT 100MHz high speed @ 1.2V pullup"
io8_100m_ft_hs_pd_1v2  "IO8_FT 100MHz high speed @ 1.2V pulldown"
io8_100m_ft_fs_1v2  "IO8_FT 100MHz fast speed @ 1.2V"
io8_100m_ft_fs_pu_1v2  "IO8_FT 100MHz fast speed @ 1.2V pullup"
io8_100m_ft_fs_pd_1v2  "IO8_FT 100MHz fast speed @ 1.2V pulldown"
io8_100m_ft_ms_1v2  "IO8_FT 100MHz med speed @ 1.2V"
io8_100m_ft_ms_pu_1v2  "IO8_FT 100MHz med speed @ 1.2V pullup"
io8_100m_ft_ms_pd_1v2  "IO8_FT 100MHz med speed @ 1.2V pulldown"
io8_100m_ft_ls_1v2  "IO8_FT 100MHz low speed @ 1.2V"
io8_100m_ft_ls_pu_1v2  "IO8_FT 100MHz low speed @ 1.2V pullup"
io8_100m_ft_ls_pd_1v2  "IO8_FT 100MHz low speed @ 1.2V pulldown"
io8_100m_ft_hs_1v8  "IO8_FT 100MHz high speed @ 1.8V"
io8_100m_ft_hs_pu_1v8  "IO8_FT 100MHz high speed @ 1.8V pullup"
io8_100m_ft_hs_pd_1v8  "IO8_FT 100MHz high speed @ 1.8V pulldown"
io8_100m_ft_fs_1v8  "IO8_FT 100MHz fast speed @ 1.8V"
io8_100m_ft_fs_pu_1v8  "IO8_FT 100MHz fast speed @ 1.8V pullup"
io8_100m_ft_fs_pd_1v8  "IO8_FT 100MHz fast speed @ 1.8V pulldown"
io8_100m_ft_ms_1v8  "IO8_FT 100MHz med speed @ 1.8V"
io8_100m_ft_ms_pu_1v8  "IO8_FT 100MHz med speed @ 1.8V pullup"
io8_100m_ft_ms_pd_1v8  "IO8_FT 100MHz med speed @ 1.8V pulldown"
io8_100m_ft_ls_1v8  "IO8_FT 100MHz low speed @ 1.8V"
io8_100m_ft_ls_pu_1v8  "IO8_FT 100MHz low speed @ 1.8V pullup"
io8_100m_ft_ls_pd_1v8  "IO8_FT 100MHz low speed @ 1.8V pulldown"
io8_100m_ft_hs_3v3  "IO8_FT 100MHz high speed @ 3.3V"
io8_100m_ft_hs_pu_3v3  "IO8_FT 100MHz high speed @ 3.3V pullup"
io8_100m_ft_hs_pd_3v3  "IO8_FT 100MHz high speed @ 3.3V pulldown"
io8_100m_ft_fs_3v3  "IO8_FT 100MHz fast speed @ 3.3V"
io8_100m_ft_fs_pu_3v3  "IO8_FT 100MHz fast speed @ 3.3V pullup"
io8_100m_ft_fs_pd_3v3  "IO8_FT 100MHz fast speed @ 3.3V pulldown"
io8_100m_ft_ms_3v3  "IO8_FT 100MHz med speed @ 3.3V"
io8_100m_ft_ms_pu_3v3  "IO8_FT 100MHz med speed @ 3.3V pullup"
io8_100m_ft_ms_pd_3v3  "IO8_FT 100MHz med speed @ 3.3V pulldown"
io8_100m_ft_ls_3v3  "IO8_FT 100MHz low speed @ 3.3V"
io8_100m_ft_ls_pu_3v3  "IO8_FT 100MHz low speed @ 3.3V pullup"
io8_100m_ft_ls_pd_3v3  "IO8_FT 100MHz low speed @ 3.3V pulldown"
io8_100m_i2c_ft_1v2  "IO8_FT 100MHz I2C @ 1.2V"
io8_100m_i2c_ft_pu_1v2  "IO8_FT 100MHz I2C @ 1.2V pullup"
io8_100m_i2c_ft_pd_1v2  "IO8_FT 100MHz I2C @ 1.2V pulldown"
io8_100m_i2c_ft_1v8  "IO8_FT 100MHz I2C @ 1.8V"
io8_100m_i2c_ft_pu_1v8  "IO8_FT 100MHz I2C @ 1.8V pullup"
io8_100m_i2c_ft_pd_1v8  "IO8_FT 100MHz I2C @ 1,8V pulldown"
io8_100m_i2c_ft_3v3  "IO8_FT 100MHz I2C @ 3.3V"
io8_100m_i2c_ft_pu_3v3  "IO8_FT 100MHz I2C HSLV @ 3.3V pullup"
io8_100m_i2c_ft_pd_3v3  "IO8_FT 100MHz I2C @ 3.3V pulldown"
[Model Selector] io8_100m_tamp_ft
io8_100m_ft_hs_1v2  "IO8_FT 100MHz high speed @ 1.2V"
io8_100m_ft_hs_pu_1v2  "IO8_FT 100MHz high speed @ 1.2V pullup"
io8_100m_ft_hs_pd_1v2  "IO8_FT 100MHz high speed @ 1.2V pulldown"
io8_100m_ft_fs_1v2  "IO8_FT 100MHz fast speed @ 1.2V"
io8_100m_ft_fs_pu_1v2  "IO8_FT 100MHz fast speed @ 1.2V pullup"
io8_100m_ft_fs_pd_1v2  "IO8_FT 100MHz fast speed @ 1.2V pulldown"
io8_100m_ft_ms_1v2  "IO8_FT 100MHz med speed @ 1.2V"
io8_100m_ft_ms_pu_1v2  "IO8_FT 100MHz med speed @ 1.2V pullup"
io8_100m_ft_ms_pd_1v2  "IO8_FT 100MHz med speed @ 1.2V pulldown"
io8_100m_ft_ls_1v2  "IO8_FT 100MHz low speed @ 1.2V"
io8_100m_ft_ls_pu_1v2  "IO8_FT 100MHz low speed @ 1.2V pullup"
io8_100m_ft_ls_pd_1v2  "IO8_FT 100MHz low speed @ 1.2V pulldown"
io8_100m_ft_hs_1v8  "IO8_FT 100MHz high speed @ 1.8V"
io8_100m_ft_hs_pu_1v8  "IO8_FT 100MHz high speed @ 1.8V pullup"
io8_100m_ft_hs_pd_1v8  "IO8_FT 100MHz high speed @ 1.8V pulldown"
io8_100m_ft_fs_1v8  "IO8_FT 100MHz fast speed @ 1.8V"
io8_100m_ft_fs_pu_1v8  "IO8_FT 100MHz fast speed @ 1.8V pullup"
io8_100m_ft_fs_pd_1v8  "IO8_FT 100MHz fast speed @ 1.8V pulldown"
io8_100m_ft_ms_1v8  "IO8_FT 100MHz med speed @ 1.8V"
io8_100m_ft_ms_pu_1v8  "IO8_FT 100MHz med speed @ 1.8V pullup"
io8_100m_ft_ms_pd_1v8  "IO8_FT 100MHz med speed @ 1.8V pulldown"
io8_100m_ft_ls_1v8  "IO8_FT 100MHz low speed @ 1.8V"
io8_100m_ft_ls_pu_1v8  "IO8_FT 100MHz low speed @ 1.8V pullup"
io8_100m_ft_ls_pd_1v8  "IO8_FT 100MHz low speed @ 1.8V pulldown"
io8_100m_ft_hs_3v3  "IO8_FT 100MHz high speed @ 3.3V"
io8_100m_ft_hs_pu_3v3  "IO8_FT 100MHz high speed @ 3.3V pullup"
io8_100m_ft_hs_pd_3v3  "IO8_FT 100MHz high speed @ 3.3V pulldown"
io8_100m_ft_fs_3v3  "IO8_FT 100MHz fast speed @ 3.3V"
io8_100m_ft_fs_pu_3v3  "IO8_FT 100MHz fast speed @ 3.3V pullup"
io8_100m_ft_fs_pd_3v3  "IO8_FT 100MHz fast speed @ 3.3V pulldown"
io8_100m_ft_ms_3v3  "IO8_FT 100MHz med speed @ 3.3V"
io8_100m_ft_ms_pu_3v3  "IO8_FT 100MHz med speed @ 3.3V pullup"
io8_100m_ft_ms_pd_3v3  "IO8_FT 100MHz med speed @ 3.3V pulldown"
io8_100m_ft_ls_3v3  "IO8_FT 100MHz low speed @ 3.3V"
io8_100m_ft_ls_pu_3v3  "IO8_FT 100MHz low speed @ 3.3V pullup"
io8_100m_ft_ls_pd_3v3  "IO8_FT 100MHz low speed @ 3.3V pulldown"
io8_ft_v33_hs_1v2  "IO8_FT_V33 high speed @ 1.2V"
io8_ft_v33_hs_pu_1v2  "IO8_FT_V33 high speed @ 1.2V pullup"
io8_ft_v33_hs_pd_1v2  "IO8_FT_V33 high speed @ 1.2V pulldown"
io8_ft_v33_fs_1v2  "IO8_FT_V33 fast speed @ 1.2V"
io8_ft_v33_fs_pu_1v2  "IO8_FT_V33 fast speed @ 1.2V pullup"
io8_ft_v33_fs_pd_1v2  "IO8_FT_V33 fast speed @ 1.2V pulldown"
io8_ft_v33_ms_1v2  "IO8_FT_V33 med speed @ 1.2V"
io8_ft_v33_ms_pu_1v2  "IO8_FT_V33 med speed @ 1.2V pullup"
io8_ft_v33_ms_pd_1v2  "IO8_FT_V33 med speed @ 1.2V pulldown"
io8_ft_v33_ls_1v2  "IO8_FT_V33 low speed @ 1.2V"
io8_ft_v33_ls_pu_1v2  "IO8_FT_V33 low speed @ 1.2V pullup"
io8_ft_v33_ls_pd_1v2  "IO8_FT_V33 low speed @ 1.2V pulldown"
io8_ft_v33_hs_1v8  "IO8_FT_V33 high speed @ 1.8V"
io8_ft_v33_hs_pu_1v8  "IO8_FT_V33 high speed @ 1.8V pullup"
io8_ft_v33_hs_pd_1v8  "IO8_FT_V33 high speed @ 1.8V pulldown"
io8_ft_v33_fs_1v8  "IO8_FT_V33 fast speed @ 1.8V"
io8_ft_v33_fs_pu_1v8  "IO8_FT_V33 fast speed @ 1.8V pullup"
io8_ft_v33_fs_pd_1v8  "IO8_FT_V33 fast speed @ 1.8V pulldown"
io8_ft_v33_ms_1v8  "IO8_FT_V33 med speed @ 1.8V"
io8_ft_v33_ms_pu_1v8  "IO8_FT_V33 med speed @ 1.8V pullup"
io8_ft_v33_ms_pd_1v8  "IO8_FT_V33 med speed @ 1.8V pulldown"
io8_ft_v33_ls_1v8  "IO8_FT_V33 low speed @ 1.8V"
io8_ft_v33_ls_pu_1v8  "IO8_FT_V33 low speed @ 1.8V pullup"
io8_ft_v33_ls_pd_1v8  "IO8_FT_V33 low speed @ 1.8V pulldown"
io8_ft_v33_hs_3v3  "IO8_FT_V33 high speed @ 3.3V"
io8_ft_v33_hs_pu_3v3  "IO8_FT_V33 high speed @ 3.3V pullup"
io8_ft_v33_hs_pd_3v3  "IO8_FT_V33 high speed @ 3.3V pulldown"
io8_ft_v33_fs_3v3  "IO8_FT_V33 fast speed @ 3.3V"
io8_ft_v33_fs_pu_3v3  "IO8_FT_V33 fast speed @ 3.3V pullup"
io8_ft_v33_fs_pd_3v3  "IO8_FT_V33 fast speed @ 3.3V pulldown"
io8_ft_v33_ms_3v3  "IO8_FT_V33 med speed @ 3.3V"
io8_ft_v33_ms_pu_3v3  "IO8_FT_V33 med speed @ 3.3V pullup"
io8_ft_v33_ms_pd_3v3  "IO8_FT_V33 med speed @ 3.3V pulldown"
io8_ft_v33_ls_3v3  "IO8_FT_V33 low speed @ 3.3V"
io8_ft_v33_ls_pu_3v3  "IO8_FT_V33 low speed @ 3.3V pullup"
io8_ft_v33_ls_pd_3v3  "IO8_FT_V33 low speed @ 3.3V pulldown"
[Model Selector] io8_usb_ft
io8_100m_ft_hs_1v2  "IO8_FT 100MHz high speed @ 1.2V"
io8_100m_ft_hs_pu_1v2  "IO8_FT 100MHz high speed @ 1.2V pullup"
io8_100m_ft_hs_pd_1v2  "IO8_FT 100MHz high speed @ 1.2V pulldown"
io8_100m_ft_fs_1v2  "IO8_FT 100MHz fast speed @ 1.2V"
io8_100m_ft_fs_pu_1v2  "IO8_FT 100MHz fast speed @ 1.2V pullup"
io8_100m_ft_fs_pd_1v2  "IO8_FT 100MHz fast speed @ 1.2V pulldown"
io8_100m_ft_ms_1v2  "IO8_FT 100MHz med speed @ 1.2V"
io8_100m_ft_ms_pu_1v2  "IO8_FT 100MHz med speed @ 1.2V pullup"
io8_100m_ft_ms_pd_1v2  "IO8_FT 100MHz med speed @ 1.2V pulldown"
io8_100m_ft_ls_1v2  "IO8_FT 100MHz low speed @ 1.2V"
io8_100m_ft_ls_pu_1v2  "IO8_FT 100MHz low speed @ 1.2V pullup"
io8_100m_ft_ls_pd_1v2  "IO8_FT 100MHz low speed @ 1.2V pulldown"
io8_100m_ft_hs_1v8  "IO8_FT 100MHz high speed @ 1.8V"
io8_100m_ft_hs_pu_1v8  "IO8_FT 100MHz high speed @ 1.8V pullup"
io8_100m_ft_hs_pd_1v8  "IO8_FT 100MHz high speed @ 1.8V pulldown"
io8_100m_ft_fs_1v8  "IO8_FT 100MHz fast speed @ 1.8V"
io8_100m_ft_fs_pu_1v8  "IO8_FT 100MHz fast speed @ 1.8V pullup"
io8_100m_ft_fs_pd_1v8  "IO8_FT 100MHz fast speed @ 1.8V pulldown"
io8_100m_ft_ms_1v8  "IO8_FT 100MHz med speed @ 1.8V"
io8_100m_ft_ms_pu_1v8  "IO8_FT 100MHz med speed @ 1.8V pullup"
io8_100m_ft_ms_pd_1v8  "IO8_FT 100MHz med speed @ 1.8V pulldown"
io8_100m_ft_ls_1v8  "IO8_FT 100MHz low speed @ 1.8V"
io8_100m_ft_ls_pu_1v8  "IO8_FT 100MHz low speed @ 1.8V pullup"
io8_100m_ft_ls_pd_1v8  "IO8_FT 100MHz low speed @ 1.8V pulldown"
io8_100m_ft_hs_3v3  "IO8_FT 100MHz high speed @ 3.3V"
io8_100m_ft_hs_pu_3v3  "IO8_FT 100MHz high speed @ 3.3V pullup"
io8_100m_ft_hs_pd_3v3  "IO8_FT 100MHz high speed @ 3.3V pulldown"
io8_100m_ft_fs_3v3  "IO8_FT 100MHz fast speed @ 3.3V"
io8_100m_ft_fs_pu_3v3  "IO8_FT 100MHz fast speed @ 3.3V pullup"
io8_100m_ft_fs_pd_3v3  "IO8_FT 100MHz fast speed @ 3.3V pulldown"
io8_100m_ft_ms_3v3  "IO8_FT 100MHz med speed @ 3.3V"
io8_100m_ft_ms_pu_3v3  "IO8_FT 100MHz med speed @ 3.3V pullup"
io8_100m_ft_ms_pd_3v3  "IO8_FT 100MHz med speed @ 3.3V pulldown"
io8_100m_ft_ls_3v3  "IO8_FT 100MHz low speed @ 3.3V"
io8_100m_ft_ls_pu_3v3  "IO8_FT 100MHz low speed @ 3.3V pullup"
io8_100m_ft_ls_pd_3v3  "IO8_FT 100MHz low speed @ 3.3V pulldown"
io8_usb_fs_3v3  "IOUSB fast speed @ 3.3V"
io8_usb_fs_pu1_3v3  "IO8USB fast speed @ 3.3V pullup1"
io8_usb_fs_pd1_3v3  "IOUSB fast speed @ 3.3V pulldown1"
io8_usb_ls_3v3  "IOUSB low speed @ 3.3V"
io8_usb_ls_pu1_3v3  "IOUSB low speed @ 3.3V pullup1"
io8_usb_ls_pd1_3v3  "IOUSB low speed @ 3.3V pulldown1"
io8_usb_fs_pu2_3v3  "IOUSB fast speed @ 3.3V pullup2"
io8_usb_fs_pd2_3v3  "IOUSB fast speed @ 3.3V pulldown2"
io8_usb_ls_pu2_3v3  "IOUSB low speed @ 3.3V pullup2"
io8_usb_ls_pd2_3v3  "IOUSB low speed @ 3.3V pulldown2"
[Model Selector] io8_166m_hslv_ft
io8_166m_ft_hs_1v2  "IO8_FT 166MHz high speed @ 1.2V"
io8_166m_ft_hs_pu_1v2  "IO8_FT 166MHz high speed @ 1.2V pullup"
io8_166m_ft_hs_pd_1v2  "IO8_FT 166MHz high speed @ 1.2V pulldown"
io8_166m_ft_fs_1v2  "IO8_FT 166MHz fast speed @ 1.2V"
io8_166m_ft_fs_pu_1v2  "IO8_FT 166MHz fast speed @ 1.2V pullup"
io8_166m_ft_fs_pd_1v2  "IO8_FT 166MHz fast speed @ 1.2V pulldown"
io8_166m_ft_ms_1v2  "IO8_FT 166MHz med speed @ 1.2V"
io8_166m_ft_ms_pu_1v2  "IO8_FT 166MHz med speed @ 1.2V pullup"
io8_166m_ft_ms_pd_1v2  "IO8_FT 166MHz med speed @ 1.2V pulldown"
io8_166m_ft_ls_1v2  "IO8_FT 166MHz low speed @ 1.2V"
io8_166m_ft_ls_pu_1v2  "IO8_FT 166MHz low speed @ 1.2V pullup"
io8_166m_ft_ls_pd_1v2  "IO8_FT 166MHz low speed @ 1.2V pulldown"
io8_166m_ft_hs_1v8  "IO8_FT 166MHz high speed @ 1.8V"
io8_166m_ft_hs_pu_1v8  "IO8_FT 166MHz high speed @ 1.8V pullup"
io8_166m_ft_hs_pd_1v8  "IO8_FT 166MHz high speed @ 1.8V pulldown"
io8_166m_ft_fs_1v8  "IO8_FT 166MHz fast speed @ 1.8V"
io8_166m_ft_fs_pu_1v8  "IO8_FT 166MHz fast speed @ 1.8V pullup"
io8_166m_ft_fs_pd_1v8  "IO8_FT 166MHz fast speed @ 1.8V pulldown"
io8_166m_ft_ms_1v8  "IO8_FT 166MHz med speed @ 1.8V"
io8_166m_ft_ms_pu_1v8  "IO8_FT 166MHz med speed @ 1.8V pullup"
io8_166m_ft_ms_pd_1v8  "IO8_FT 166MHz med speed @ 1.8V pulldown"
io8_166m_ft_ls_1v8  "IO8_FT 166MHz low speed @ 1.8V"
io8_166m_ft_ls_pu_1v8  "IO8_FT 166MHz low speed @ 1.8V pullup"
io8_166m_ft_ls_pd_1v8  "IO8_FT 166MHz low speed @ 1.8V pulldown"
io8_166m_ft_hs_3v3  "IO8_FT 166MHz high speed @ 3.3V"
io8_166m_ft_hs_pu_3v3  "IO8_FT 166MHz high speed @ 3.3V pullup"
io8_166m_ft_hs_pd_3v3  "IO8_FT 166MHz high speed @ 3.3V pulldown"
io8_166m_ft_fs_3v3  "IO8_FT 166MHz fast speed @ 3.3V"
io8_166m_ft_fs_pu_3v3  "IO8_FT 166MHz fast speed @ 3.3V pullup"
io8_166m_ft_fs_pd_3v3  "IO8_FT 166MHz fast speed @ 3.3V pulldown"
io8_166m_ft_ms_3v3  "IO8_FT 166MHz med speed @ 3.3V"
io8_166m_ft_ms_pu_3v3  "IO8_FT 166MHz med speed @ 3.3V pullup"
io8_166m_ft_ms_pd_3v3  "IO8_FT 166MHz med speed @ 3.3V pulldown"
io8_166m_ft_ls_3v3  "IO8_FT 166MHz low speed @ 3.3V"
io8_166m_ft_ls_pu_3v3  "IO8_FT 166MHz low speed @ 3.3V pullup"
io8_166m_ft_ls_pd_3v3  "IO8_FT 166MHz low speed @ 3.3V pulldown"
io8_166m_hslv_ft_hs_1v2  "IO8_FT 166MHz HSLV high speed @ 1.2V"
io8_166m_hslv_ft_hs_pu_1v2  "IO8_FT 166MHz HSLV high speed @ 1.2V pullup"
io8_166m_hslv_ft_hs_pd_1v2  "IO8_FT 166MHz HSLV high speed @ 1.2V pulldown"
io8_166m_hslv_ft_fs_1v2  "IO8_FT 166MHz HSLV fast speed @ 1.2V"
io8_166m_hslv_ft_fs_pu_1v2  "IO8_FT 166MHz HSLV fast speed @ 1.2V pullup"
io8_166m_hslv_ft_fs_pd_1v2  "IO8_FT 166MHz HSLV fast speed @ 1.2V pulldown"
io8_166m_hslv_ft_ms_1v2  "IO8_FT 166MHz HSLV med speed @ 1.2V"
io8_166m_hslv_ft_ms_pu_1v2  "IO8_FT 166MHz HSLV med speed @ 1.2V pullup"
io8_166m_hslv_ft_ms_pd_1v2  "IO8_FT 166MHz HSLV med speed @ 1.2V pulldown"
io8_166m_hslv_ft_ls_1v2  "IO8_FT 166MHz HSLV low speed @ 1.2V"
io8_166m_hslv_ft_ls_pu_1v2  "IO8_FT 166MHz HSLV low speed @ 1.2V pullup"
io8_166m_hslv_ft_ls_pd_1v2  "IO8_FT 166MHz HSLV low speed @ 1.2V pulldown"
io8_166m_hslv_ft_hs_1v8  "IO8_FT 166MHz HSLV high speed @ 1.8V"
io8_166m_hslv_ft_hs_pu_1v8  "IO8_FT 166MHz HSLV high speed @ 1.8V pullup"
io8_166m_hslv_ft_hs_pd_1v8  "IO8_FT 166MHz HSLV high speed @ 1.8V pulldown"
io8_166m_hslv_ft_fs_1v8  "IO8_FT 166MHz HSLV fast speed @ 1.8V"
io8_166m_hslv_ft_fs_pu_1v8  "IO8_FT 166MHz HSLV fast speed @ 1.8V pullup"
io8_166m_hslv_ft_fs_pd_1v8  "IO8_FT 166MHz HSLV fast speed @ 1.8V pulldown"
io8_166m_hslv_ft_ms_1v8  "IO8_FT 166MHz HSLV med speed @ 1.8V"
io8_166m_hslv_ft_ms_pu_1v8  "IO8_FT 166MHz HSLV med speed @ 1.8V pullup"
io8_166m_hslv_ft_ms_pd_1v8  "IO8_FT 166MHz HSLV med speed @ 1.8V pulldown"
io8_166m_hslv_ft_ls_1v8  "IO8_FT 166MHz HSLV low speed @ 1.8V"
io8_166m_hslv_ft_ls_pu_1v8  "IO8_FT 166MHz HSLV low speed @ 1.8V pullup"
io8_166m_hslv_ft_ls_pd_1v8  "IO8_FT 166MHz HSLV low speed @ 1.8V pulldown"
io8_166m_hslv_ft_hs_2v5  "IO8_FT 166MHz HSLV high speed @ 2.5V"
io8_166m_hslv_ft_hs_pu_2v5  "IO8_FT 166MHz HSLV high speed @ 2.5V pullup"
io8_166m_hslv_ft_hs_pd_2v5  "IO8_FT 166MHz HSLV high speed @ 2.5V pulldown"
io8_166m_hslv_ft_fs_2v5  "IO8_FT 166MHz HSLV fast speed @ 2.5V"
io8_166m_hslv_ft_fs_pu_2v5  "IO8_FT 166MHz HSLV fast speed @ 2.5V pullup"
io8_166m_hslv_ft_fs_pd_2v5  "IO8_FT 166MHz HSLV fast speed @ 2.5V pulldown"
io8_166m_hslv_ft_ms_2v5  "IO8_FT 166MHz HSLV med speed @ 2.5V"
io8_166m_hslv_ft_ms_pu_2v5  "IO8_FT 166MHz HSLV med speed @ 2.5V pullup"
io8_166m_hslv_ft_ms_pd_2v5  "IO8_FT 166MHz HSLV med speed @ 2.5V pulldown"
io8_166m_hslv_ft_ls_2v5  "IO8_FT 166MHz HSLV low speed @ 2.5V"
io8_166m_hslv_ft_ls_pu_2v5  "IO8_FT 166MHz HSLV low speed @ 2.5V pullup"
io8_166m_hslv_ft_ls_pd_2v5  "IO8_FT 166MHz HSLV low speed @ 2.5V pulldown"
[Model Selector] io8_166m_hslv_i2c_ft
io8_166m_ft_hs_1v2  "IO8_FT 166MHz high speed @ 1.2V"
io8_166m_ft_hs_pu_1v2  "IO8_FT 166MHz high speed @ 1.2V pullup"
io8_166m_ft_hs_pd_1v2  "IO8_FT 166MHz high speed @ 1.2V pulldown"
io8_166m_ft_fs_1v2  "IO8_FT 166MHz fast speed @ 1.2V"
io8_166m_ft_fs_pu_1v2  "IO8_FT 166MHz fast speed @ 1.2V pullup"
io8_166m_ft_fs_pd_1v2  "IO8_FT 166MHz fast speed @ 1.2V pulldown"
io8_166m_ft_ms_1v2  "IO8_FT 166MHz med speed @ 1.2V"
io8_166m_ft_ms_pu_1v2  "IO8_FT 166MHz med speed @ 1.2V pullup"
io8_166m_ft_ms_pd_1v2  "IO8_FT 166MHz med speed @ 1.2V pulldown"
io8_166m_ft_ls_1v2  "IO8_FT 166MHz low speed @ 1.2V"
io8_166m_ft_ls_pu_1v2  "IO8_FT 166MHz low speed @ 1.2V pullup"
io8_166m_ft_ls_pd_1v2  "IO8_FT 166MHz low speed @ 1.2V pulldown"
io8_166m_ft_hs_1v8  "IO8_FT 166MHz high speed @ 1.8V"
io8_166m_ft_hs_pu_1v8  "IO8_FT 166MHz high speed @ 1.8V pullup"
io8_166m_ft_hs_pd_1v8  "IO8_FT 166MHz high speed @ 1.8V pulldown"
io8_166m_ft_fs_1v8  "IO8_FT 166MHz fast speed @ 1.8V"
io8_166m_ft_fs_pu_1v8  "IO8_FT 166MHz fast speed @ 1.8V pullup"
io8_166m_ft_fs_pd_1v8  "IO8_FT 166MHz fast speed @ 1.8V pulldown"
io8_166m_ft_ms_1v8  "IO8_FT 166MHz med speed @ 1.8V"
io8_166m_ft_ms_pu_1v8  "IO8_FT 166MHz med speed @ 1.8V pullup"
io8_166m_ft_ms_pd_1v8  "IO8_FT 166MHz med speed @ 1.8V pulldown"
io8_166m_ft_ls_1v8  "IO8_FT 166MHz low speed @ 1.8V"
io8_166m_ft_ls_pu_1v8  "IO8_FT 166MHz low speed @ 1.8V pullup"
io8_166m_ft_ls_pd_1v8  "IO8_FT 166MHz low speed @ 1.8V pulldown"
io8_166m_ft_hs_3v3  "IO8_FT 166MHz high speed @ 3.3V"
io8_166m_ft_hs_pu_3v3  "IO8_FT 166MHz high speed @ 3.3V pullup"
io8_166m_ft_hs_pd_3v3  "IO8_FT 166MHz high speed @ 3.3V pulldown"
io8_166m_ft_fs_3v3  "IO8_FT 166MHz fast speed @ 3.3V"
io8_166m_ft_fs_pu_3v3  "IO8_FT 166MHz fast speed @ 3.3V pullup"
io8_166m_ft_fs_pd_3v3  "IO8_FT 166MHz fast speed @ 3.3V pulldown"
io8_166m_ft_ms_3v3  "IO8_FT 166MHz med speed @ 3.3V"
io8_166m_ft_ms_pu_3v3  "IO8_FT 166MHz med speed @ 3.3V pullup"
io8_166m_ft_ms_pd_3v3  "IO8_FT 166MHz med speed @ 3.3V pulldown"
io8_166m_ft_ls_3v3  "IO8_FT 166MHz low speed @ 3.3V"
io8_166m_ft_ls_pu_3v3  "IO8_FT 166MHz low speed @ 3.3V pullup"
io8_166m_ft_ls_pd_3v3  "IO8_FT 166MHz low speed @ 3.3V pulldown"
io8_166m_hslv_ft_hs_1v2  "IO8_FT 166MHz HSLV high speed @ 1.2V"
io8_166m_hslv_ft_hs_pu_1v2  "IO8_FT 166MHz HSLV high speed @ 1.2V pullup"
io8_166m_hslv_ft_hs_pd_1v2  "IO8_FT 166MHz HSLV high speed @ 1.2V pulldown"
io8_166m_hslv_ft_fs_1v2  "IO8_FT 166MHz HSLV fast speed @ 1.2V"
io8_166m_hslv_ft_fs_pu_1v2  "IO8_FT 166MHz HSLV fast speed @ 1.2V pullup"
io8_166m_hslv_ft_fs_pd_1v2  "IO8_FT 166MHz HSLV fast speed @ 1.2V pulldown"
io8_166m_hslv_ft_ms_1v2  "IO8_FT 166MHz HSLV med speed @ 1.2V"
io8_166m_hslv_ft_ms_pu_1v2  "IO8_FT 166MHz HSLV med speed @ 1.2V pullup"
io8_166m_hslv_ft_ms_pd_1v2  "IO8_FT 166MHz HSLV med speed @ 1.2V pulldown"
io8_166m_hslv_ft_ls_1v2  "IO8_FT 166MHz HSLV low speed @ 1.2V"
io8_166m_hslv_ft_ls_pu_1v2  "IO8_FT 166MHz HSLV low speed @ 1.2V pullup"
io8_166m_hslv_ft_ls_pd_1v2  "IO8_FT 166MHz HSLV low speed @ 1.2V pulldown"
io8_166m_hslv_ft_hs_1v8  "IO8_FT 166MHz HSLV high speed @ 1.8V"
io8_166m_hslv_ft_hs_pu_1v8  "IO8_FT 166MHz HSLV high speed @ 1.8V pullup"
io8_166m_hslv_ft_hs_pd_1v8  "IO8_FT 166MHz HSLV high speed @ 1.8V pulldown"
io8_166m_hslv_ft_fs_1v8  "IO8_FT 166MHz HSLV fast speed @ 1.8V"
io8_166m_hslv_ft_fs_pu_1v8  "IO8_FT 166MHz HSLV fast speed @ 1.8V pullup"
io8_166m_hslv_ft_fs_pd_1v8  "IO8_FT 166MHz HSLV fast speed @ 1.8V pulldown"
io8_166m_hslv_ft_ms_1v8  "IO8_FT 166MHz HSLV med speed @ 1.8V"
io8_166m_hslv_ft_ms_pu_1v8  "IO8_FT 166MHz HSLV med speed @ 1.8V pullup"
io8_166m_hslv_ft_ms_pd_1v8  "IO8_FT 166MHz HSLV med speed @ 1.8V pulldown"
io8_166m_hslv_ft_ls_1v8  "IO8_FT 166MHz HSLV low speed @ 1.8V"
io8_166m_hslv_ft_ls_pu_1v8  "IO8_FT 166MHz HSLV low speed @ 1.8V pullup"
io8_166m_hslv_ft_ls_pd_1v8  "IO8_FT 166MHz HSLV low speed @ 1.8V pulldown"
io8_166m_hslv_ft_hs_2v5  "IO8_FT 166MHz HSLV high speed @ 2.5V"
io8_166m_hslv_ft_hs_pu_2v5  "IO8_FT 166MHz HSLV high speed @ 2.5V pullup"
io8_166m_hslv_ft_hs_pd_2v5  "IO8_FT 166MHz HSLV high speed @ 2.5V pulldown"
io8_166m_hslv_ft_fs_2v5  "IO8_FT 166MHz HSLV fast speed @ 2.5V"
io8_166m_hslv_ft_fs_pu_2v5  "IO8_FT 166MHz HSLV fast speed @ 2.5V pullup"
io8_166m_hslv_ft_fs_pd_2v5  "IO8_FT 166MHz HSLV fast speed @ 2.5V pulldown"
io8_166m_hslv_ft_ms_2v5  "IO8_FT 166MHz HSLV med speed @ 2.5V"
io8_166m_hslv_ft_ms_pu_2v5  "IO8_FT 166MHz HSLV med speed @ 2.5V pullup"
io8_166m_hslv_ft_ms_pd_2v5  "IO8_FT 166MHz HSLV med speed @ 2.5V pulldown"
io8_166m_hslv_ft_ls_2v5  "IO8_FT 166MHz HSLV low speed @ 2.5V"
io8_166m_hslv_ft_ls_pu_2v5  "IO8_FT 166MHz HSLV low speed @ 2.5V pullup"
io8_166m_hslv_ft_ls_pd_2v5  "IO8_FT 166MHz HSLV low speed @ 2.5V pulldown"
io8_166m_i2c_ft_1v2  "IO8_FT 166MHz I2C @ 1.2V"
io8_166m_i2c_ft_pu_1v2  "IO8_FT 166MHz I2C @ 1.2V pullup"
io8_166m_i2c_ft_pd_1v2  "IO8_FT 166MHz I2C @ 1.2V pulldown"
io8_166m_i2c_ft_1v8  "IO8_FT 166MHz I2C @ 1.8V"
io8_166m_i2c_ft_pu_1v8  "IO8_FT 166MHz I2C @ 1.8V pullup"
io8_166m_i2c_ft_pd_1v8  "IO8_FT 166MHz I2C @ 1,8V pulldown"
io8_166m_i2c_ft_3v3  "IO8_FT 166MHz I2C @ 3.3V"
io8_166m_i2c_ft_pu_3v3  "IO8_FT 166MHz I2C HSLV @ 3.3V pullup"
io8_166m_i2c_ft_pd_3v3  "IO8_FT 166MHz I2C @ 3.3V pulldown"
[Model Selector] io8_100m_ft_v33
io8_ft_v33_hs_1v2  "IO8_FT_V33 high speed @ 1.2V"
io8_ft_v33_hs_pu_1v2  "IO8_FT_V33 high speed @ 1.2V pullup"
io8_ft_v33_hs_pd_1v2  "IO8_FT_V33 high speed @ 1.2V pulldown"
io8_ft_v33_fs_1v2  "IO8_FT_V33 fast speed @ 1.2V"
io8_ft_v33_fs_pu_1v2  "IO8_FT_V33 fast speed @ 1.2V pullup"
io8_ft_v33_fs_pd_1v2  "IO8_FT_V33 fast speed @ 1.2V pulldown"
io8_ft_v33_ms_1v2  "IO8_FT_V33 med speed @ 1.2V"
io8_ft_v33_ms_pu_1v2  "IO8_FT_V33 med speed @ 1.2V pullup"
io8_ft_v33_ms_pd_1v2  "IO8_FT_V33 med speed @ 1.2V pulldown"
io8_ft_v33_ls_1v2  "IO8_FT_V33 low speed @ 1.2V"
io8_ft_v33_ls_pu_1v2  "IO8_FT_V33 low speed @ 1.2V pullup"
io8_ft_v33_ls_pd_1v2  "IO8_FT_V33 low speed @ 1.2V pulldown"
io8_ft_v33_hs_1v8  "IO8_FT_V33 high speed @ 1.8V"
io8_ft_v33_hs_pu_1v8  "IO8_FT_V33 high speed @ 1.8V pullup"
io8_ft_v33_hs_pd_1v8  "IO8_FT_V33 high speed @ 1.8V pulldown"
io8_ft_v33_fs_1v8  "IO8_FT_V33 fast speed @ 1.8V"
io8_ft_v33_fs_pu_1v8  "IO8_FT_V33 fast speed @ 1.8V pullup"
io8_ft_v33_fs_pd_1v8  "IO8_FT_V33 fast speed @ 1.8V pulldown"
io8_ft_v33_ms_1v8  "IO8_FT_V33 med speed @ 1.8V"
io8_ft_v33_ms_pu_1v8  "IO8_FT_V33 med speed @ 1.8V pullup"
io8_ft_v33_ms_pd_1v8  "IO8_FT_V33 med speed @ 1.8V pulldown"
io8_ft_v33_ls_1v8  "IO8_FT_V33 low speed @ 1.8V"
io8_ft_v33_ls_pu_1v8  "IO8_FT_V33 low speed @ 1.8V pullup"
io8_ft_v33_ls_pd_1v8  "IO8_FT_V33 low speed @ 1.8V pulldown"
io8_ft_v33_hs_3v3  "IO8_FT_V33 high speed @ 3.3V"
io8_ft_v33_hs_pu_3v3  "IO8_FT_V33 high speed @ 3.3V pullup"
io8_ft_v33_hs_pd_3v3  "IO8_FT_V33 high speed @ 3.3V pulldown"
io8_ft_v33_fs_3v3  "IO8_FT_V33 fast speed @ 3.3V"
io8_ft_v33_fs_pu_3v3  "IO8_FT_V33 fast speed @ 3.3V pullup"
io8_ft_v33_fs_pd_3v3  "IO8_FT_V33 fast speed @ 3.3V pulldown"
io8_ft_v33_ms_3v3  "IO8_FT_V33 med speed @ 3.3V"
io8_ft_v33_ms_pu_3v3  "IO8_FT_V33 med speed @ 3.3V pullup"
io8_ft_v33_ms_pd_3v3  "IO8_FT_V33 med speed @ 3.3V pulldown"
io8_ft_v33_ls_3v3  "IO8_FT_V33 low speed @ 3.3V"
io8_ft_v33_ls_pu_3v3  "IO8_FT_V33 low speed @ 3.3V pullup"
io8_ft_v33_ls_pd_3v3  "IO8_FT_V33 low speed @ 3.3V pulldown"
[Define Package Model]  455-wlcsp-72-100mhz-230421
[Manufacturer]  Unknown
[OEM]  Unknown
[Description]  None
[Number Of Pins]  72
[Pin Numbers]
| Pin Num   Terminal Name
E14 | NRST
H15 | PA0
E12 | PA1
F11 | PA2
G12 | PA3
H13 | PA4
E10 | PA5
H11 | PA6
J12 | PA7
E4 | PA8
F9 | PA9
E6 | PA10
C2 | PA11
C4 | PA12
D5 | PA13
E8 | PA14
D7 | PA15
G10 | PB0
G8 | PB1
J10 | PB2
C10 | PB3
A10 | PB4
D11 | PB5
B11 | PB6
D13 | PB7
C12 | PB8
H9 | PB10
G4 | PB13
G2 | PB14
H1 | PB15
F13 | PC1
C14 | PC13
C16 | PC14-OSC32_IN
D15 | PC15-OSC32_OUT
G6 | PG2
H7 | PG3
F1 | PG4
F3 | PG5
F5 | PG6
F7 | PG7
E2 | PG8
B5 | PG9
A4 | PG10
C6 | PG11
D9 | PG12
C8 | PG13
A6 | PG14
B9 | PG15
E16 | PH0-OSC_IN
F15 | PH1-OSC_OUT
A12 | PH3-BOOT0
J4 | VDD11
A14 | VDD11
B15 | VBAT
B1 | VDDUSB
A2 | VDD
A16 | VDD
J2 | VDD
J14 | VDD
G14 | VDDA
D1 | VDDIO2
A8 | VDDIO2
J6 | VDDSMPS
J8 | VLXSMPS
B3 | VSS
B7 | VSS
B13 | VSS
D3 | VSS
H3 | VSS
J16 | VSS
G16 | VSSA
H5 | VSSSMPS
[Model Data]
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[End Model Data]
[End Package Model]
| Models and submodels in the file (208): io8_100m_ft_hs_1v2 (I/O), io8_100m_ft_hs_pu_1v2 (I/O), io8_100m_ft_hs_pd_1v2 (I/O), io8_100m_ft_fs_1v2 (I/O), io8_100m_ft_fs_pu_1v2 (I/O), io8_100m_ft_fs_pd_1v2 (I/O), io8_100m_ft_ms_1v2 (I/O), io8_100m_ft_ms_pu_1v2 (I/O), io8_100m_ft_ms_pd_1v2 (I/O), io8_100m_ft_ls_1v2 (I/O), io8_100m_ft_ls_pu_1v2 (I/O), io8_100m_ft_ls_pd_1v2 (I/O), io8_100m_ft_hs_1v8 (I/O), io8_100m_ft_hs_pu_1v8 (I/O), io8_100m_ft_hs_pd_1v8 (I/O), io8_100m_ft_fs_1v8 (I/O), io8_100m_ft_fs_pu_1v8 (I/O), io8_100m_ft_fs_pd_1v8 (I/O), io8_100m_ft_ms_1v8 (I/O), io8_100m_ft_ms_pu_1v8 (I/O), io8_100m_ft_ms_pd_1v8 (I/O), io8_100m_ft_ls_1v8 (I/O), io8_100m_ft_ls_pu_1v8 (I/O), io8_100m_ft_ls_pd_1v8 (I/O), io8_100m_ft_hs_3v3 (I/O), io8_100m_ft_hs_pu_3v3 (I/O), io8_100m_ft_hs_pd_3v3 (I/O), io8_100m_ft_fs_3v3 (I/O), io8_100m_ft_fs_pu_3v3 (I/O), io8_100m_ft_fs_pd_3v3 (I/O), io8_100m_ft_ms_3v3 (I/O), io8_100m_ft_ms_pu_3v3 (I/O), io8_100m_ft_ms_pd_3v3 (I/O), io8_100m_ft_ls_3v3 (I/O), io8_100m_ft_ls_pu_3v3 (I/O), io8_100m_ft_ls_pd_3v3 (I/O), io8_100m_hslv_ft_hs_1v2 (I/O), io8_100m_hslv_ft_hs_pu_1v2 (I/O), io8_100m_hslv_ft_hs_pd_1v2 (I/O), io8_100m_hslv_ft_fs_1v2 (I/O), io8_100m_hslv_ft_fs_pu_1v2 (I/O), io8_100m_hslv_ft_fs_pd_1v2 (I/O), io8_100m_hslv_ft_ms_1v2 (I/O), io8_100m_hslv_ft_ms_pu_1v2 (I/O), io8_100m_hslv_ft_ms_pd_1v2 (I/O), io8_100m_hslv_ft_ls_1v2 (I/O), io8_100m_hslv_ft_ls_pu_1v2 (I/O), io8_100m_hslv_ft_ls_pd_1v2 (I/O), io8_100m_hslv_ft_hs_1v8 (I/O), io8_100m_hslv_ft_hs_pu_1v8 (I/O), io8_100m_hslv_ft_hs_pd_1v8 (I/O), io8_100m_hslv_ft_fs_1v8 (I/O), io8_100m_hslv_ft_fs_pu_1v8 (I/O), io8_100m_hslv_ft_fs_pd_1v8 (I/O), io8_100m_hslv_ft_ms_1v8 (I/O), io8_100m_hslv_ft_ms_pu_1v8 (I/O), io8_100m_hslv_ft_ms_pd_1v8 (I/O), io8_100m_hslv_ft_ls_1v8 (I/O), io8_100m_hslv_ft_ls_pu_1v8 (I/O), io8_100m_hslv_ft_ls_pd_1v8 (I/O), io8_100m_hslv_ft_hs_2v5 (I/O), io8_100m_hslv_ft_hs_pu_2v5 (I/O), io8_100m_hslv_ft_hs_pd_2v5 (I/O), io8_100m_hslv_ft_fs_2v5 (I/O), io8_100m_hslv_ft_fs_pu_2v5 (I/O), io8_100m_hslv_ft_fs_pd_2v5 (I/O), io8_100m_hslv_ft_ms_2v5 (I/O), io8_100m_hslv_ft_ms_pu_2v5 (I/O), io8_100m_hslv_ft_ms_pd_2v5 (I/O), io8_100m_hslv_ft_ls_2v5 (I/O), io8_100m_hslv_ft_ls_pu_2v5 (I/O), io8_100m_hslv_ft_ls_pd_2v5 (I/O), io8_166m_ft_hs_1v2 (I/O), io8_166m_ft_hs_pu_1v2 (I/O), io8_166m_ft_hs_pd_1v2 (I/O), io8_166m_ft_fs_1v2 (I/O), io8_166m_ft_fs_pu_1v2 (I/O), io8_166m_ft_fs_pd_1v2 (I/O), io8_166m_ft_ms_1v2 (I/O), io8_166m_ft_ms_pu_1v2 (I/O)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
